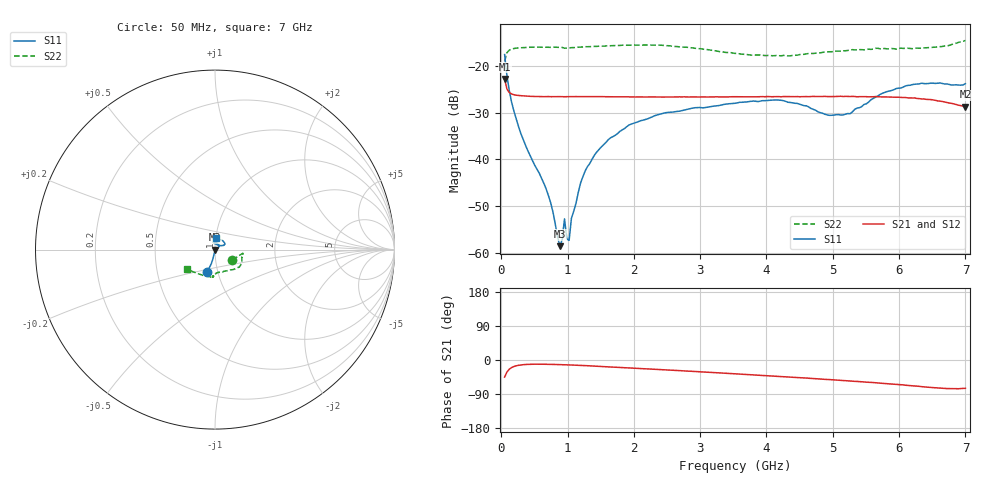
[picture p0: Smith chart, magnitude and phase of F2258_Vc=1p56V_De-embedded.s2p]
! Integrated Device Technology
! Corporate Headquarters
! 6024 Silver Creek Valley Road
! San Jose, CA 95138  USA
! Phone:  1-408-284-8200
! Toll Free:  1-800-223-1366
! Webpage:  http://www.idt.com/
! Timing and RF Division
! 515 Groton Road, Suite 102
! Westford, MA 01886-6024
! Device:  F2258
! Description: Voltage Variable RF Attenuator
! Frequency:  50.0 -  6000.00 MHz
! Package:  3x3 mm Thin QFN Plastic Package: 16 pin
! Ports:  2 RF, 2 DC
!  Pin  1  = NC
!  Pin  2  = NC
!  Pin  3  = RF2  = Port 2
!  Pin  4  = GND
!  Pin  5  = Vdd
!  Pin  6  = NC
!  Pin  7  = VCTRL
!  Pin  8  = NC
!  Pin  9  = GND
!  Pin 10  = RF1  = Port 1
!  Pin 11  = NC
!  Pin 12  = NC
!  Pin 13  = NC
!  Pin 14  = NC
!  Pin 15  = NC
!  Pin 16  = NC
! Vcntrl:  1.560 Volts
! Vdd:  +3.300 Volts
! Current:  1.161 mA
! Data:  The device was measured on a the F2258 evaluation board which has
!  individual transmission lines to the RF pins.  Data was collected
!  using a calibrated network analyzer.  The evaluation board was
!  de-embedded using a TRL calibration technique.
!  The reference plane is the edge of the package pin.
! Misc:  SN 10
!  Action Tracker AT0285
! Date Measured:  2014-12-10
! Date:  2016-01-13  MJV
! Note:
!  Integrated Device Technology supplies this data as a sample of measured
!  data at the package pin for this product.  Your particular data for this
!  product may vary.
!  Data was taken at 25 degrees C.
!  Integrated Device Technology reserves the right to change this data at anytime.
!Freq_(GHz)  S11M_(dB)  S11P_(deg)  S21M_(dB)  S21P_(deg)  S12M_(dB)  S12P_(deg)  S22M_(dB)  S22P_(deg)
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# GHz S dB R 50
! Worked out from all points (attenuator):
!   201 points, 50 MHz to 7 GHz, reference 50 ohm
!   highest |S21| = -22.80 dB at 50 MHz (marker M1); lowest = -28.7 dB at 7 GHz (marker M2)
!   lowest |S11| = -58.5 dB at 884 MHz (marker M3), VSWR 1.00, Z = 50.1 - j0.0336 ohm
!   |S11| at or under -10 dB: start of sweep to end of sweep
!   |S22| runs from -19.0 to -14.6 dB; largest |S21 - S12| = 0.00048
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0.05  -17.57 -109.0  -22.80 -45.0  -22.79 -45.0  -18.99 -30.3
0.1195  -25.21 -103.0  -25.68 -24.4  -25.65 -24.4  -16.64 -10.3
0.189  -29.60 -103.1  -26.16 -17.2  -26.15 -17.2  -16.29 -7.9
0.36275  -36.87 -103.3  -26.45 -11.9  -26.43 -11.9  -16.05 -8.1
0.71025  -47.69 -91.1  -26.54 -11.4  -26.54 -11.4  -16.01 -12.1
0.884  -58.54 -16.5  -26.56 -12.2  -26.62 -12.2  -16.03 -15.2
0.91875  -57.09 12.3  -26.57 -12.4  -26.62 -12.4  -16.04 -15.8
0.9535  -52.69 -102.0  -26.59 -12.6  -26.62 -12.6  -16.21 -15.6
0.98825  -56.97 -94.9  -26.57 -12.8  -26.63 -12.8  -16.18 -16.5
1.023  -57.30 -35.8  -26.57 -13.0  -26.62 -13.0  -16.13 -17.1
1.05775  -52.60 -13.5  -26.57 -13.2  -26.63 -13.2  -16.09 -17.4
1.2315  -43.66 16.1  -26.57 -14.5  -26.59 -14.5  -15.93 -20.1
1.40525  -39.07 18.0  -26.55 -16.2  -26.58 -16.1  -15.83 -22.4
1.61375  -35.77 22.1  -26.59 -18.1  -26.61 -18.1  -15.69 -25.6
2.37825  -30.36 41.4  -26.65 -25.1  -26.70 -25.1  -15.58 -35.6
3.525  -27.99 88.6  -26.58 -36.5  -26.60 -36.5  -17.32 -59.6
4.22  -27.34 104.0  -26.60 -43.7  -26.61 -43.7  -17.83 -80.1
4.7065  -29.28 94.0  -26.51 -48.9  -26.52 -48.9  -17.34 -89.6
5.2625  -30.21 49.6  -26.54 -55.3  -26.57 -55.2  -16.59 -93.8
5.85325  -25.37 26.7  -26.66 -63.0  -26.67 -63.0  -16.36 -96.2
6.33975  -23.69 32.8  -27.07 -70.4  -27.05 -70.3  -16.23 -107.1
7  -23.79 83.5  -28.70 -74.6  -28.80 -74.6  -14.55 -145.1
